DATA_BLOCK DB_AID
TITLE = Analog Inputs DST
//Analog Input Destination DATA Block
VERSION : 0.1
  STRUCT
K04HJA10CR001XQ01 : UAI_DST; //HOØÁK È.1 - VELIKOST PLAMENE 4-20mA
K04HJA20CR001XQ01 : UAI_DST; //HOØÁK È.2 - VELIKOST PLAMENE 4-20mA
K04HJA30CR001XQ01 : UAI_DST; //HOØÁK È.3 - VELIKOST PLAMENE 4-20mA
K04HJA40CR001XQ01 : UAI_DST; //HOØÁK È.4 - VELIKOST PLAMENE 4-20mA
K04HHG36AS001XQ01 : UAI_DST; //HOØÁK È.1 - POLOHA KLAPKY PLYNU
K04HHL11AS010XQ01 : UAI_DST; //HOØÁK È.1 - POLOHA KLAPKY VZDUCHU
K04HHG37AS001XQ01 : UAI_DST; //HOØÁK È.2 - POLOHA KLAPKY PLYNU
K04HHL71AS010XQ01 : UAI_DST; //HOØÁK È.2 - POLOHA KLAPKY VZDUCHU
K04HHG38AS001XQ01 : UAI_DST; //HOØÁK È.3 - POLOHA KLAPKY PLYNU
K04HHL51AS010XQ01 : UAI_DST; //HOØÁK È.3 - POLOHA KLAPKY VZDUCHU
K04HHG39AS001XQ01 : UAI_DST; //HOØÁK È.4 - POLOHA KLAPKY PLYNU
K04HHL31AS010XQ01 : UAI_DST; //HOØÁK È.4 - POLOHA KLAPKY VZDUCHU
PIW536 : UAI_DST; //REZERVA
PIW538 : UAI_DST; //REZERVA
PIW540 : UAI_DST; //REZERVA
PIW542 : UAI_DST; //REZERVA
END_STRUCT ;
BEGIN

END_DATA_BLOCK

